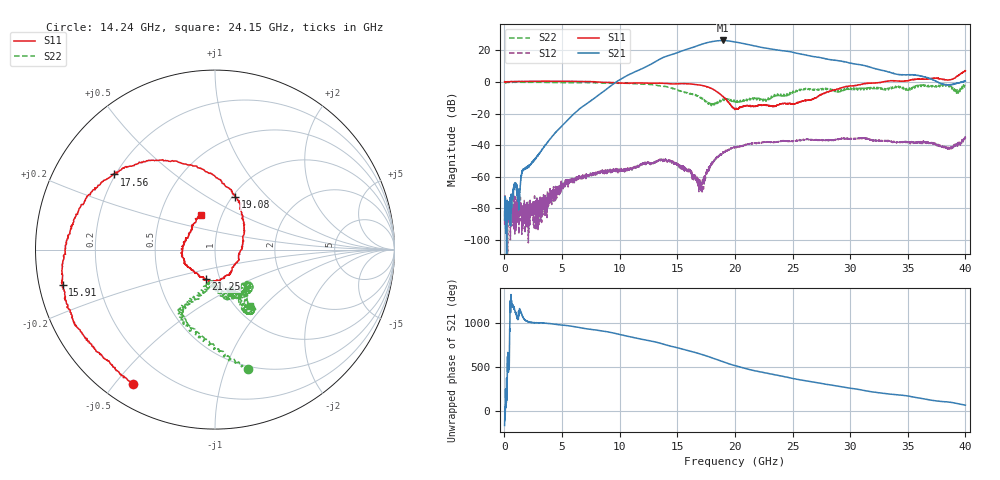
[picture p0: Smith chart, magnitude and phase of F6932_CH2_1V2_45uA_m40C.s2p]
!Keysight Technologies,M9807A,MY58100526,A.15.20.05
!Date: Tuesday, August 01, 2023 10:03:23
!Correction: S11(Cdelta 2-Port  )
!S21(Cdelta 2-Port  )
!S12(Cdelta 2-Port  )
!S22(Cdelta 2-Port  )
!S2P File: Measurements: S11, S21, S12, S22:
# Hz S  dB  R 50
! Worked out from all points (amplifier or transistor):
!   4000 points, 10 MHz to 40 GHz, reference 50 ohm
!   highest |S21| = 26.2 dB at 18.99 GHz (marker M1)
!   |S21| within 3 dB of that: 16.89 GHz to 21.37 GHz (4.48 GHz wide, 23.4 % of centre)
!   unconditionally stable (mu >= 1): 8.02 GHz to 31.1 GHz; 31.12744 GHz to 31.2226 GHz; 31.81779 GHz to 31.90773 GHz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
!   at 6.67 GHz: K = -18.17, MSG = 22.1 dB, |S12| = -60.4 dB
!   at 20.01 GHz: K = 2.94, MAG = 25.6 dB, |S12| = -41.1 dB
!   at 40 GHz: K = -33.64, MSG = 17.7 dB, |S12| = -34.9 dB
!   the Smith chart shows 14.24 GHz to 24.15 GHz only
!   S11 on the Smith chart (normalised r, x): 14.24 GHz: 0.09, -0.56; 15.91 GHz: 0.07, -0.11; 17.56 GHz: 0.20, +0.32; 19.08 GHz: 1.03, +0.67; 21.25 GHz: 0.86, -0.29; 24.15 GHz: 0.79, +0.32
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1e7  0.10 178.6  -87.25 -159.9  -81.46 -59.9  -0.61 178.2
6.68e9  0.22 68.8  -16.09 -140.4  -59.68 138.1  -0.47 65.9
1.093e10  -0.81 -37.6  5.01 118.7  -54.71 100.4  -0.99 -10.0
1.334e10  -0.87 -91.2  13.77 53.7  -49.73 60.9  -2.33 -52.2
1.424e10  -1.16 -121.3  16.62 20.3  -50.24 25.9  -3.21 -74.8
1.591e10  -1.19 -166.8  20.77 -35.0  -55.83 -7.7  -7.21 -111.0
1.682e10  -1.88 169.4  23.04 -67.0  -63.46 -75.0  -9.00 -116.6
1.756e10  -3.10 143.2  24.73 -97.4  -55.70 149.0  -13.52 -105.9
1.827e10  -5.38 113.6  25.75 -129.3  -49.03 120.7  -13.67 -93.8
1.899e10  -9.39 73.8  26.18 -162.8  -44.44 93.8  -10.94 -73.3
1.908e10  -10.10 68.9  26.11 -167.1  -44.67 91.5  -11.13 -76.1
1.948e10  -13.28 42.4  25.81 175.3  -42.95 77.2  -11.44 -70.8
2.001e10  -17.41 -12.9  25.21 154.2  -41.06 57.8  -12.39 -71.3
2.062e10  -15.60 -71.3  24.38 131.8  -40.49 43.5  -11.66 -66.5
2.125e10  -15.35 -107.9  23.37 110.9  -39.11 26.7  -10.78 -67.4
2.266e10  -14.86 -177.9  21.37 72.0  -37.89 -5.9  -11.60 -48.3
2.415e10  -13.59 112.6  19.69 34.3  -37.15 -31.8  -8.62 -58.6
2.503e10  -14.00 77.1  18.68 9.6  -37.45 -49.2  -6.07 -90.5
2.667e10  -11.25 7.6  16.17 -28.0  -36.30 -78.4  -4.45 -84.6
2.998e10  -2.59 -75.9  11.92 -99.0  -36.11 -134.0  -4.64 -115.9
3.334e10  0.53 -140.2  6.26 -164.9  -37.28 168.3  -4.75 -152.0
4e10  7.00 95.9  0.50 69.3  -34.90 44.3  -1.69 118.8
